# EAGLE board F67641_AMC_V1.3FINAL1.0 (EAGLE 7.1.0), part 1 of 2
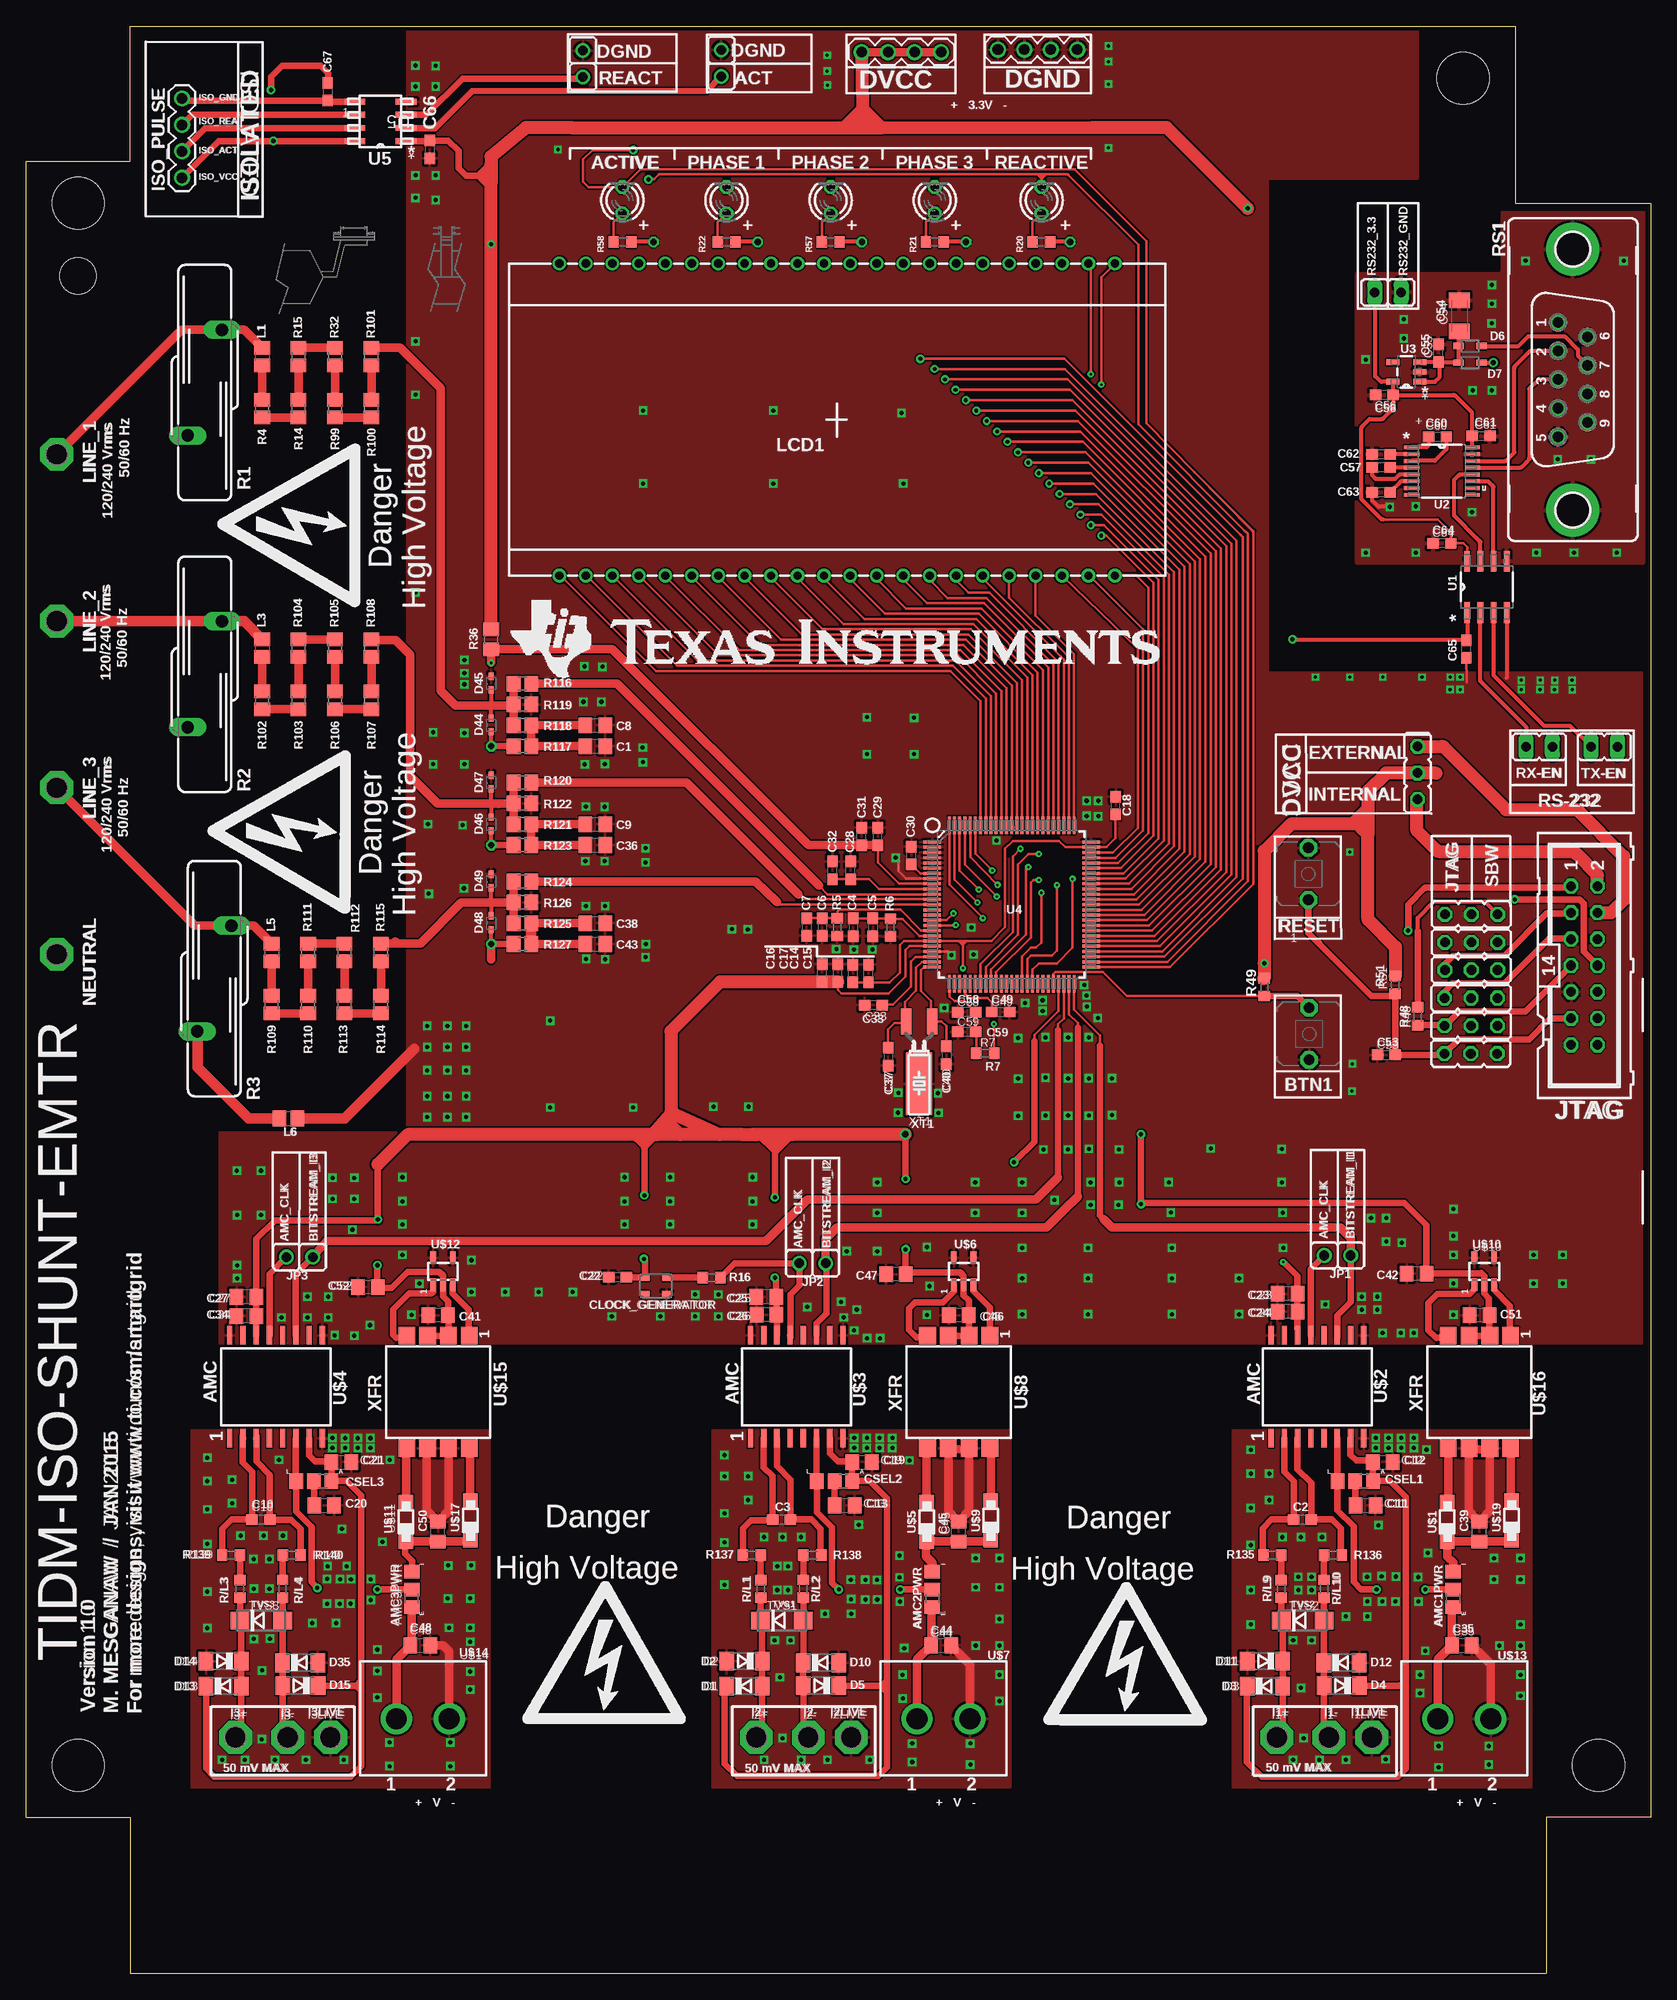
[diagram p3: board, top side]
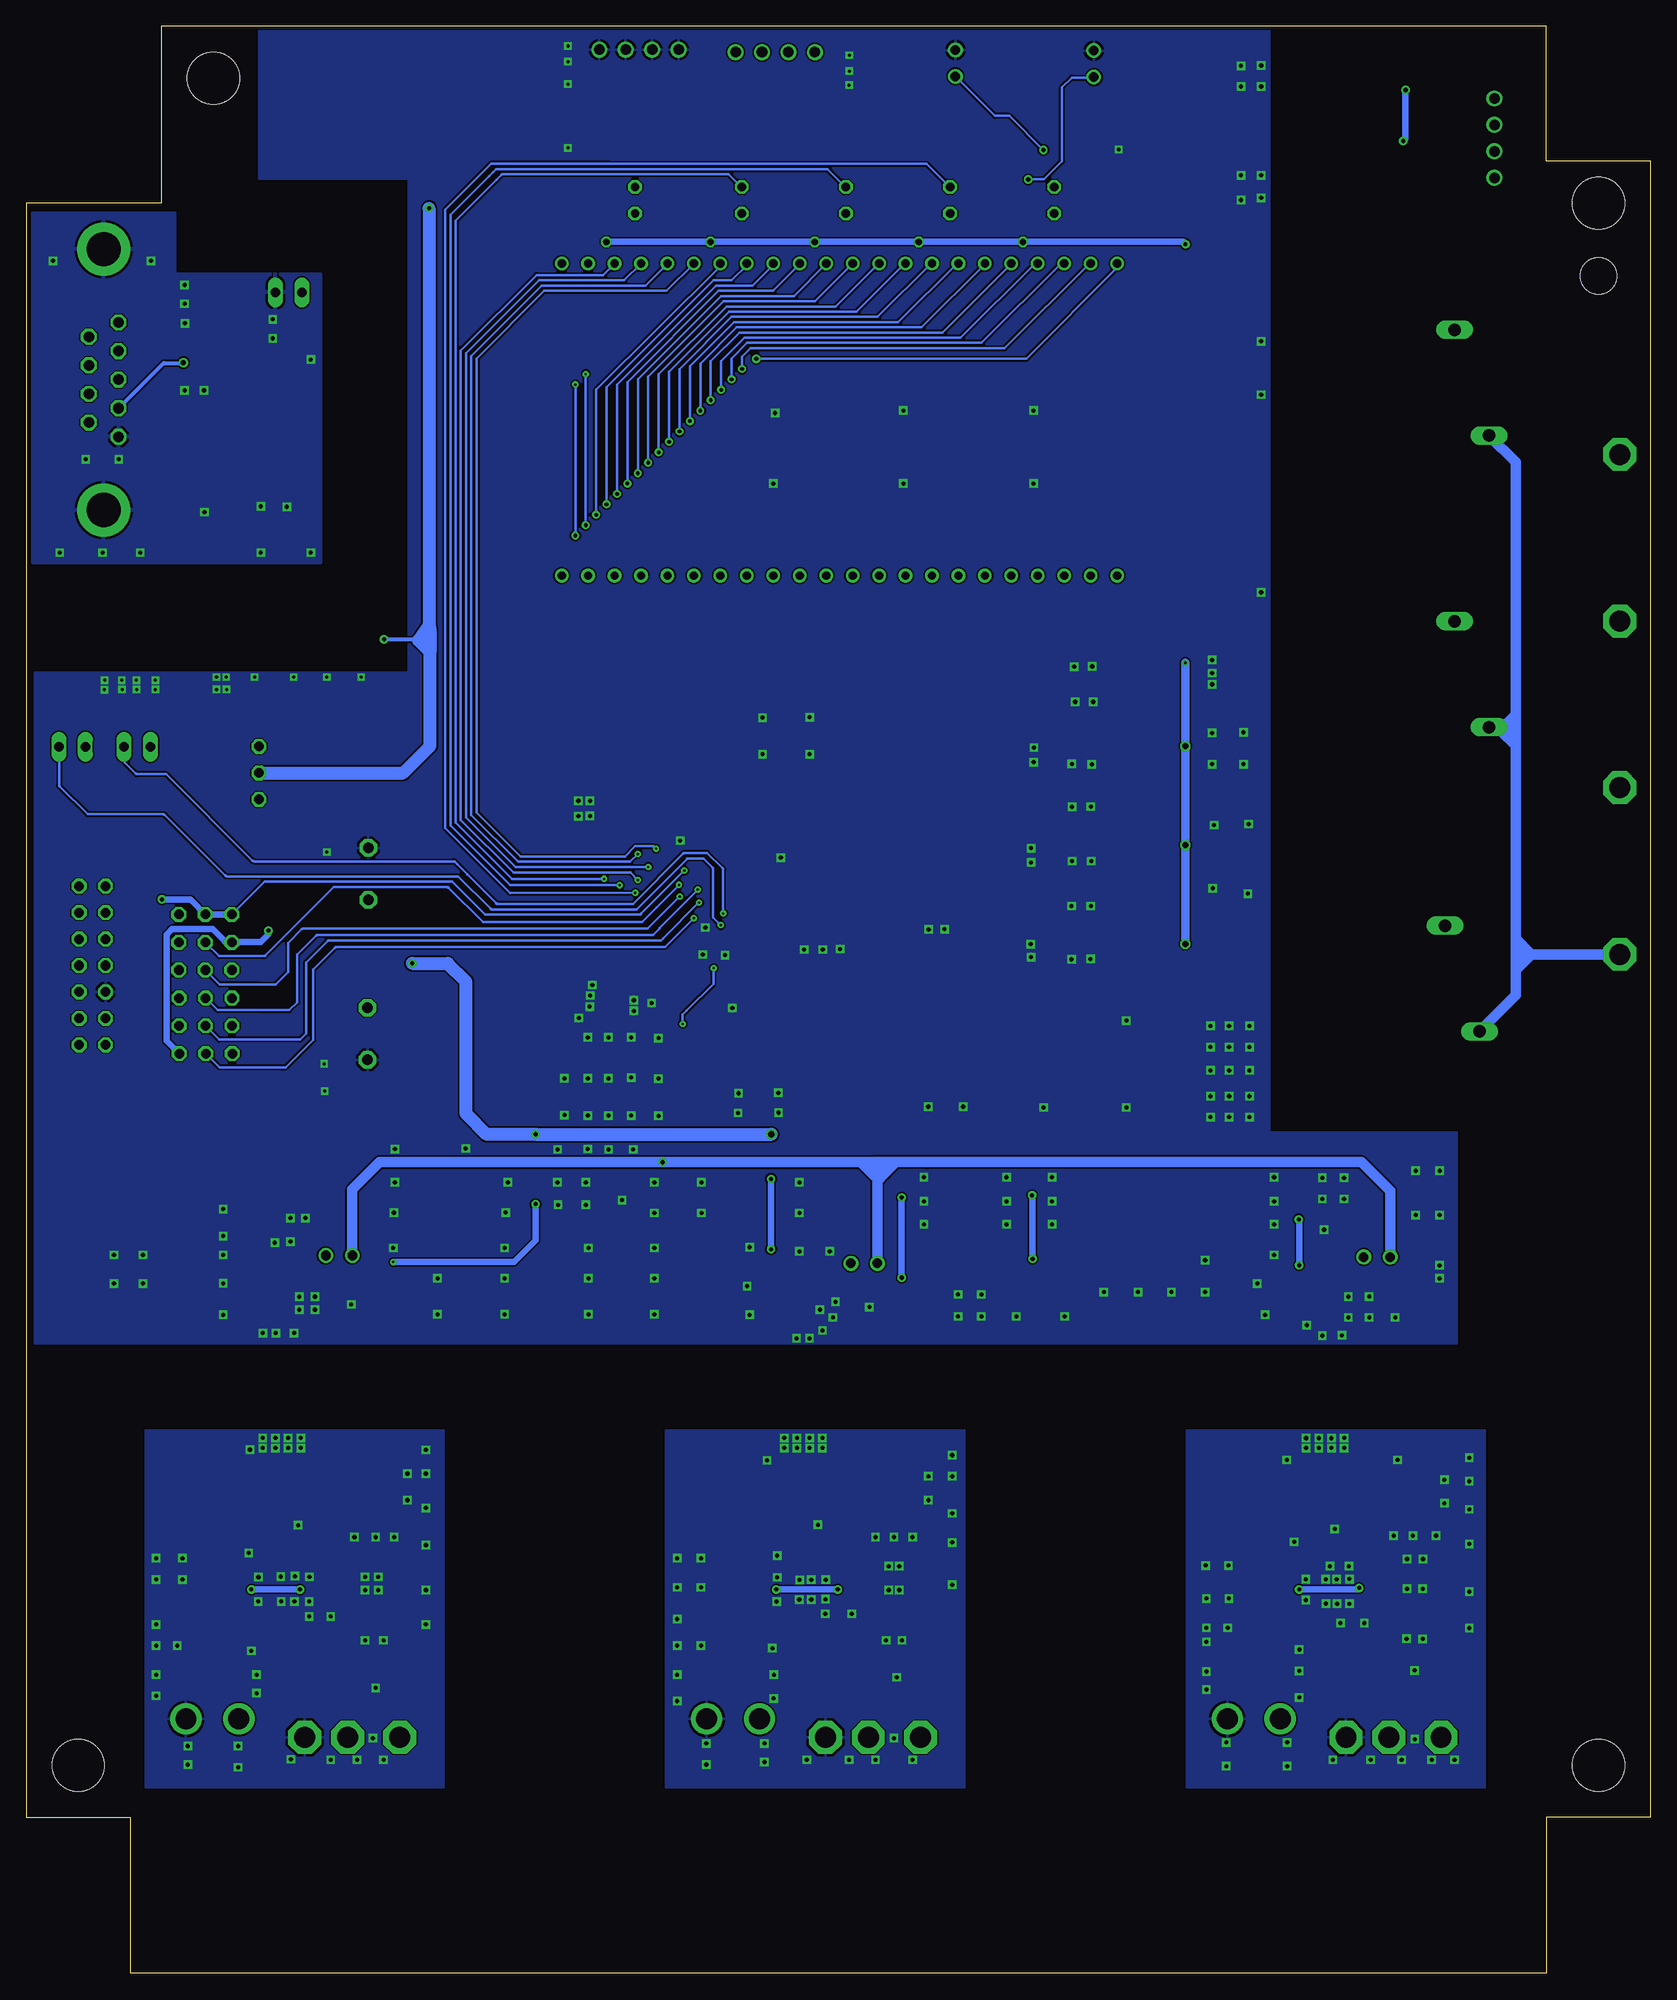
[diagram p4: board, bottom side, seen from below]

Size 156 x 187 mm. Coordinates in mm from the lower left corner, seen from the top.
Copper layers (1*16): Top 0.0356mm / dielectric 1.5011mm / Bottom 0.0356mm
Design rules "typical_4pcb *": minimum track width 10mil, minimum drill 0.2mm, track to track 6mil, track to pad 6mil, pad to pad 6mil, via to via 6mil, smd to smd 6mil, copper to edge 15mil, drill to drill 8mil, minimum pad ring 10mil, minimum via ring 8mil, stop-mask expansion 4mil, vias tented up to drill 25mil, thermal gap 10mil

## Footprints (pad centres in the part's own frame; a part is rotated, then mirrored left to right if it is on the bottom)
JP1 = drill 0.914: 1 0,-1.27; 2 0,1.27
A0R-JMP = smd 1.5 x 1.3: 1 0,1.7; 2 0,0; 3 0,-1.7
PBTH = drill 1.016 pad 1.676 octagon: 1 -0.001,0.001; 2 5.001,0.001
C0805 = smd 1.3 x 1.5: 1 -0.95,0; 2 0.95,0
C0603 = smd 1.1 x 1: 1 -0.85,0; 2 0.85,0
C1206K = smd 1.5 x 2: 1 -1.5,0; 2 1.5,0
3_PHASE_CASE = hole 5: 0,0; 146,0; 0,150; 133,162 | hole 3.5: 0,143
ASE = smd 0.9 x 0.65: 1 -1.05,-0.825; 2 1.05,-0.825; 3 1.05,0.825; 4 -1.05,0.825
SOD80C = smd 1.4 x 1.8: A 1.7,0; C -1.7,0
SOD323 = smd 1 x 0.6: 1 -1.1,0; 2 1.1,0
SOD523 = smd 0.7 x 0.5: A 0.7,0; C -0.6,0
MA04-1 = drill 1.016: 1 -3.81,0; 2 -1.27,0; 3 1.27,0; 4 3.81,0
P1-20 = drill 2.007 pad 3.15 octagon: TP 0,0
JP2 = drill 0.914 octagon: 1 -2.54,0; 2 0,0; 3 2.54,0
JP1' = drill 0.914 long: 1 0,-1.27; 2 0,1.27
ML14 = drill 0.914 octagon: 1 -7.62,-1.27; 2 -7.62,1.27; 3 -5.08,-1.27; 4 -5.08,1.27; 5 -2.54,-1.27; 6 -2.54,1.27; 7 0,-1.27; 8 0,1.27; 9 2.54,-1.27; 10 2.54,1.27; 11 5.08,-1.27; 12 5.08,1.27; 13 7.62,-1.27; 14 7.62,1.27
R0805 = smd 1.3 x 1.5: 1 -0.85,0; 2 0.85,0
TI_160SEG_LCD = drill 0.8: 1 4.826,0; 2 7.366,0; 3 9.906,0; 4 12.446,0; 5 14.986,0; 6 17.526,0; 7 20.066,0; 8 22.606,0; 9 25.146,0; 10 27.686,0; 11 30.226,0; 12 32.766,0; 13 35.306,0; 14 37.846,0; 15 40.386,0; 16 42.926,0; 17 45.466,0; 18 48.006,0; 19 50.546,0; 20 53.086,0; 21 55.626,0; 22 58.166,0; 23 58.166,29.972; 24 55.626,29.972; 29 42.926,29.972; 30 40.386,29.972; 31 37.846,29.972; 32 35.306,29.972; 33 32.766,29.972; 34 30.226,29.972; 35 27.686,29.972; 36 25.146,29.972; 37 22.606,29.972; 38 20.066,29.972; 39 17.526,29.972; 40 14.986,29.972; 41 12.446,29.972; 42 9.906,29.972; 43 7.366,29.972; 44 4.826,29.972; COM0 45.466,29.972; COM1 48.006,29.972; COM2 50.546,29.972; COM3 53.086,29.972
LED3MM = drill 0.813 octagon: A -1.27,0; K 1.27,0
S20K275 = drill 1.194 long: 1 -1.651,-5.08; 2 1.651,5.08
R0603 = smd 1 x 1.1: 1 -0.85,0; 2 0.85,0
R0805' = smd 1.3 x 1.5: 1 -0.95,0; 2 0.95,0
F09VP = drill 1.016 octagon: 1 5.486,1.422; 2 2.743,1.422; 3 0,1.422; 4 -2.743,1.422; 5 -5.486,1.422; 6 4.115,-1.422; 7 1.372,-1.422; 8 -1.372,-1.422; 9 -4.115,-1.422 | drill 3.302 pad 5.08: G1 -12.522,0; G2 12.522,0
DO214AC = smd 1.8 x 1.7: A 2.05,0; C -2.05,0
SOIC127P600X175-8N = smd 1.981 x 0.559: 1 -2.464,1.905; 2 -2.464,0.635; 3 -2.464,-0.635; 4 -2.464,-1.905; 5 2.464,-1.905; 6 2.464,-0.635; 7 2.464,0.635; 8 2.464,1.905
SOP65P640X120-16N = smd 1.473 x 0.356: 1 -2.921,2.286; 2 -2.921,1.626; 3 -2.921,0.965; 4 -2.921,0.33; 5 -2.921,-0.33; 6 -2.921,-0.965; 7 -2.921,-1.626; 8 -2.921,-2.286; 9 2.921,-2.286; 10 2.921,-1.626; 11 2.921,-0.965; 12 2.921,-0.33; 13 2.921,0.33; 14 2.921,0.965; 15 2.921,1.626; 16 2.921,2.286
SOT95P280X145-5N = smd 1.27 x 0.559: 1 -1.295,0.94; 2 -1.295,0; 3 -1.295,-0.94; 4 1.295,-0.94; 5 1.295,0.94
PZ100 = smd 1.676 x 0.279: 1 -7.62,5.994; 2 -7.62,5.512; 3 -7.62,5.004; 4 -7.62,4.496; 5 -7.62,3.988; 6 -7.62,3.505; 7 -7.62,2.997; 8 -7.62,2.489; 9 -7.62,2.007; 10 -7.62,1.499; 11 -7.62,0.991; 12 -7.62,0.508; 13 -7.62,0; 14 -7.62,-0.508; 15 -7.62,-0.991; 16 -7.62,-1.499; 17 -7.62,-2.007; 18 -7.62,-2.489; 19 -7.62,-2.997; 20 -7.62,-3.505; 21 -7.62,-3.988; 22 -7.62,-4.496; 23 -7.62,-5.004; 24 -7.62,-5.512; 25 -7.62,-5.994; 51 7.62,-5.994; 52 7.62,-5.512; 53 7.62,-5.004; 54 7.62,-4.496; 55 7.62,-3.988; 56 7.62,-3.505; 57 7.62,-2.997; 58 7.62,-2.489; 59 7.62,-2.007; 60 7.62,-1.499; 61 7.62,-0.991; 62 7.62,-0.508; 63 7.62,0; 64 7.62,0.508; 65 7.62,0.991; 66 7.62,1.499; 67 7.62,2.007; 68 7.62,2.489; 69 7.62,2.997; 70 7.62,3.505; 71 7.62,3.988; 72 7.62,4.496; 73 7.62,5.004; 74 7.62,5.512; 75 7.62,5.994 | smd 0.279 x 1.676: 26 -5.994,-7.62; 27 -5.512,-7.62; 28 -5.004,-7.62; 29 -4.496,-7.62; 30 -3.988,-7.62; 31 -3.505,-7.62; 32 -2.997,-7.62; 33 -2.489,-7.62; 34 -2.007,-7.62; 35 -1.499,-7.62; 36 -0.991,-7.62; 37 -0.508,-7.62; 38 0,-7.62; 39 0.508,-7.62; 40 0.991,-7.62; 41 1.499,-7.62; 42 2.007,-7.62; 43 2.489,-7.62; 44 2.997,-7.62; 45 3.505,-7.62; 46 3.988,-7.62; 47 4.496,-7.62; 48 5.004,-7.62; 49 5.512,-7.62; 50 5.994,-7.62; 76 5.994,7.62; 77 5.512,7.62; 78 5.004,7.62; 79 4.496,7.62; 80 3.988,7.62; 81 3.505,7.62; 82 2.997,7.62; 83 2.489,7.62; 84 2.007,7.62; 85 1.499,7.62; 86 0.991,7.62; 87 0.508,7.62; 88 0,7.62; 89 -0.508,7.62; 90 -0.991,7.62; 91 -1.499,7.62; 92 -2.007,7.62; 93 -2.489,7.62; 94 -2.997,7.62; 95 -3.505,7.62; 96 -3.988,7.62; 97 -4.496,7.62; 98 -5.004,7.62; 99 -5.512,7.62; 100 -5.994,7.62
D8 = smd 1.981 x 0.559: 1 -2.464,1.905; 2 -2.464,0.635; 3 -2.464,-0.635; 4 -2.464,-1.905; 5 2.464,-1.905; 6 2.464,-0.635; 7 2.464,0.635; 8 2.464,1.905
SOD123 = smd 1.4 x 1.4: A 1.9,0; C -1.9,0
SOIC-16DW = smd 1.778 x 0.508: AGND -5.029,-3.988; AINN -5.029,2.362; AINP -5.029,3.632; AVDD -5.029,-2.718; CLKIN 4.851,1.092; DGND1 4.851,-3.988; DGND2 4.851,4.902; DOUT 4.851,-1.448; DVDD 4.851,2.362; LDO_IN -5.029,-1.448; NC1 -5.029,4.902; NC2 -5.029,1.092; NC3 -5.029,-0.178; NC5 4.851,-2.718; NC6 4.851,-0.178; NC7 4.851,3.632
SOT23-DBV = smd 0.55 x 1.2: 1 -0.95,-1.3; 2 0,-1.3; 3 0.95,-1.3; 4 0.95,1.3; 5 -0.95,1.3
TERMINALBLOCK5.08 = drill 2: 1 -2.54,0; 2 2.54,0
DA2303-AL = smd 1.7 x 1.6: 1 -5.01,3.37; 2 -5.01,1.37; 3 -5.01,-0.63; 4 -5.01,-2.63; 5 5.79,-2.63; 6 5.79,-0.63; 7 5.79,1.37; 8 5.79,3.37
CM200T = smd 1 x 2.5: P1 -1.25,-5; P2 1.25,-5 | smd 2.5 x 6: P3 0,1

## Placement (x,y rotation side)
ACT  [JP1]  66.76,183.43 180 top
AMC1PWR  0R-JUMPA  [A0R-JMP]  137.04,36.87 180 top
AMC2PWR  0R-JUMPA  [A0R-JMP]  87.04,36.87 180 top
AMC3PWR  0R-JUMPA  [A0R-JMP]  37.04,36.87 180 top
BTN1  [PBTH]  123.22,87.73 90 top
C1  100nF  [C0805]  54.67,117.85 0 top
C2  5600pF  [C0603]  122.56,43.6 0 top
C3  5600pF  [C0603]  72.56,43.6 0 top
C4  4.7uF  [C0603]  79.43,100.45 270 top
C5  100nF  [C0603]  81.31,100.46 270 top
C6  4.7uF  [C0603]  76.46,100.5 270 top
C7  100nF  [C0603]  74.96,100.5 270 top
C8  10uF  [C0805]  54.67,119.85 0 top
C9  100nF  [C0805]  54.67,110.35 0 top
C10  5600pF  [C0603]  22.56,43.6 0 top
C11  0.1u  [C0805]  128.63,44.95 0 top
C12  4.7uF  [C0805]  130.28,49.11 0 top
C13  0.1u  [C0805]  78.63,44.95 0 top
C14  4.7uF  [C0603]  79.4,96.02 90 top
C15  100nF  [C0603]  80.9,96.02 90 top
C16  4.7uF  [C0603]  76.46,96.06 90 top
C17  100nF  [C0603]  77.96,96.06 90 top
C18  0.1uF  [C0603]  104.65,112.14 90 top
C19  4.7uF  [C0805]  80.28,49.11 0 top
C20  0.1u  [C0805]  28.63,44.95 0 top
C21  4.7uF  [C0805]  30.28,49.11 0 top
C22  0.01uF  [C0603]  56.81,66.86 180 top
C23  0.1u  [C0805]  121.14,65.27 180 top
C24  2.2uF  [C0805]  121.14,63.56 180 top
C25  0.1u  [C0805]  71.09,64.96 180 top
C26  2.2uF  [C0805]  71.11,63.26 180 top
C27  0.1u  [C0805]  21.16,64.96 180 top
C28  100nF  [C0603]  79.19,105.93 90 top
C29  4.7uF  [C0603]  81.79,109.18 90 top
C30  100nF  [C0603]  85.02,107.35 90 top
C31  100nF  [C0603]  80.24,109.18 90 top
C32  4.7uF  [C0603]  77.44,105.93 90 top
C33  470nF  [C0603]  81.38,92.98 180 top
C34  2.2uF  [C0805]  21.16,63.13 180 top
C35  10u  [C0805]  137.88,31.51 0 top
C36  10uF  [C0805]  54.67,108.35 0 top
C37  12pF  [C0603]  82.79,88.03 270 top
C38  100nF  [C0805]  54.67,100.85 0 top
C39  10u  [C0805]  139.55,42.43 90 top
C40  12pF  [C0603]  88.38,88.17 270 top
C41  10u  [C0805]  39.58,63.21 180 top
C42  0.1u  [C0805]  133.53,67.2 180 top
C43  10uF  [C0805]  54.67,98.85 0 top
C44  10u  [C0805]  87.88,31.51 0 top
C45  10u  [C0805]  89.55,42.43 90 top
C46  10u  [C0805]  89.58,63.21 180 top
C47  0.1u  [C0805]  83.53,67.15 180 top
C48  10u  [C0805]  37.88,31.51 0 top
C49  4.7uF  [C0603]  93.59,92.32 0 top
C50  10u  [C0805]  39.55,42.43 90 top
C51  10u  [C0805]  139.58,63.21 180 top
C52  0.1u  [C0805]  32.82,65.9 180 top
C53  0.1uF  [C0603]  130.64,88.2 0 top
C54  47u  [C1206K]  137.65,159.17 90 top
C55  1u  [C0603]  135.64,155.59 90 top
C56  0.1u  [C0603]  130.43,151.58 180 top
C57  0.1u  [C0603]  130.13,144.62 180 top
C58  0.47uF  [C0603]  90.33,92.32 180 top
C59  100nF  [C0603]  90.33,90.41 180 top
C60  0.1u  [C0603]  135.54,147.56 0 top
C61  0.1u  [C0603]  139.73,147.64 0 top
C62  0.1u  [C0603]  130.13,145.89 0 top
C63  0.1u  [C0603]  130.13,142.23 0 top
C64  0.1u  [C0603]  135.97,137.33 180 top
C65  0.1u  [C0603]  138.31,127.17 90 top
C66  0.1u  [C0603]  38.76,175.15 270 top
C67  0.1u  [C0603]  28.96,180.68 270 top
CASE1  3_PHASE_CASE  [3_PHASE_CASE]  5,20 0 top
CLOCK_GENERATOR  ASE  [ASE]  60.48,66.02 0 top
CSEL1  0R-JUMPA  [A0R-JMP]  127.64,47.28 270 top
CSEL2  0R-JUMPA  [A0R-JMP]  77.64,47.28 270 top
CSEL3  0R-JUMPA  [A0R-JMP]  27.64,47.28 270 top
D1  PMLL4148  [SOD80C]  68.98,27.59 0 top
D2  PMLL4148  [SOD80C]  68.98,29.99 180 top
D3  PMLL4148  [SOD80C]  118.98,27.59 0 top
D4  PMLL4148  [SOD80C]  126.35,27.64 180 top
D5  PMLL4148  [SOD80C]  76.35,27.64 180 top
D6  1N4148  [SOD323]  138.66,156.27 0 top
D7  1N4148  [SOD323]  138.66,154.67 0 top
D10  PMLL4148  [SOD80C]  76.32,29.84 0 top
D11  PMLL4148  [SOD80C]  118.98,29.99 180 top
D12  PMLL4148  [SOD80C]  126.32,29.84 0 top
D13  PMLL4148  [SOD80C]  18.98,27.59 0 top
D14  PMLL4148  [SOD80C]  18.98,29.99 180 top
D15  PMLL4148  [SOD80C]  26.35,27.64 180 top
D35  PMLL4148  [SOD80C]  26.32,29.84 0 top
D44  1N4148DO35-7  [SOD523]  44.67,119.85 90 top
D45  1N4148DO35-7  [SOD523]  44.67,123.85 90 top
D46  1N4148DO35-7  [SOD523]  44.67,110.35 90 top
D47  1N4148DO35-7  [SOD523]  44.67,114.35 90 top
D48  1N4148DO35-7  [SOD523]  44.67,100.85 90 top
D49  1N4148DO35-7  [SOD523]  44.67,104.85 90 top
DGND  [MA04-1]  97.14,184.73 0 top
DVCC  [MA04-1]  84.05,184.5 0 top
I1+  TPPAD1-20  [P1-20]  120.12,22.67 0 top
I1-  TPPAD1-20  [P1-20]  125.12,22.67 0 top
I1LIVE  TPPAD1-20  [P1-20]  129.24,22.67 0 top
I2+  TPPAD1-20  [P1-20]  70.12,22.67 0 top
I2-  TPPAD1-20  [P1-20]  75.12,22.67 0 top
I2LIVE  TPPAD1-20  [P1-20]  79.24,22.67 0 top
I3+  TPPAD1-20  [P1-20]  20.12,22.67 0 top
I3-  TPPAD1-20  [P1-20]  25.12,22.67 0 top
I3LIVE  TPPAD1-20  [P1-20]  29.24,22.67 0 top
ISO_PULSE  [MA04-1]  14.99,176.24 90 top
JP1  [JP1]  125.94,68.95 90 top
JP2  [JP1]  75.52,68.19 90 top
JP3  [JP1]  26.27,68.8 90 top
JP4  [JP2]  138.79,101.69 180 top
JP5  [JP2]  138.74,88.33 180 top
JP6  [JP2]  138.76,91 180 top
JP7  [JP2]  138.76,93.66 180 top
JP8  [JP2]  138.79,96.36 180 top
JP9  [JP2]  138.79,99 180 top
JP10  [JP2]  133.63,115.28 90 top
JP14  [JP1']  130.79,161.43 270 top
JP15  [JP1']  145.32,117.79 90 top
JP16  [JP1']  151.57,117.79 90 top
JTAG  [ML14]  149.64,96.79 270 top
L1  EXCML20A  [R0805]  22.67,155.26 270 top
L3  EXCML20A  [R0805]  22.67,127.26 270 top
L5  EXCML20A  [R0805]  23.59,98.04 270 top
L6  EXCML20A  [R0805]  25.2,82.1 0 top
LCD1  TI_160SEG_LCD  [TI_160SEG_LCD]  46.4,134.23 0 top
LED_ACT  [LED3MM]  57.27,170.27 90 top
LED_PHASE_1  [LED3MM]  67.27,170.27 90 top
LED_PHASE_2  [LED3MM]  77.27,170.27 90 top
LED_PHASE_3  [LED3MM]  87.27,170.27 90 top
LED_REACT  [LED3MM]  97.52,170.27 90 top
LINE_1  TPPAD1-20  [P1-20]  2.96,145.86 0 top
LINE_2  TPPAD1-20  [P1-20]  2.96,129.86 0 top
LINE_3  TPPAD1-20  [P1-20]  2.96,113.86 0 top
NEUTRAL  TPPAD1-20  [P1-20]  2.96,97.86 0 top
R1  S20K275  [S20K275]  17.17,152.76 0 top
R2  S20K275  [S20K275]  17.17,124.76 0 top
R3  S20K275  [S20K275]  18.09,95.54 0 top
R4  1M  [R0805]  22.67,150.26 90 top
R5  0  [R0603]  77.88,100.47 90 top
R6  0  [R0603]  83.01,100.44 90 top
R7  0  [R0603]  92.1,88.38 180 top
R14  1M  [R0805]  26.17,150.26 270 top
R15  1M  [R0805]  26.17,155.26 270 top
R16  0  [R0603]  65.83,66.81 0 top
R20  100  [R0603]  97.52,166.27 180 top
R21  100  [R0603]  87.27,166.27 180 top
R22  100  [R0603]  67.27,166.27 180 top
R32  1M  [R0805]  29.67,155.26 90 top
R36  10R  [R0805']  44.66,128.11 270 top
R48  330  [R0603]  133.63,91.91 90 top
R49  100K  [R0603]  118.91,94.71 270 top
R51  47K  [R0603]  131.47,94.93 270 top
R57  100  [R0603]  77.27,166.27 180 top
R58  100  [R0603]  57.27,166.27 180 top
R99  1M  [R0805]  29.67,150.26 90 top
R100  1M  [R0805]  33.17,150.26 270 top
R101  1M  [R0805]  33.17,155.26 270 top
R102  1M  [R0805]  22.67,122.26 90 top
R103  1M  [R0805]  26.17,122.26 270 top
R104  1M  [R0805]  26.17,127.26 270 top
R105  1M  [R0805]  29.67,127.26 90 top
R106  1M  [R0805]  29.67,122.26 90 top
R107  1M  [R0805]  33.17,122.26 270 top
R108  1M  [R0805]  33.17,127.26 270 top
R109  1M  [R0805]  23.59,93.04 90 top
R110  1M  [R0805]  27.09,93.04 270 top
R111  1M  [R0805]  27.09,98.04 270 top
R112  1M  [R0805]  30.59,98.04 90 top
R113  1M  [R0805]  30.59,93.04 90 top
R114  1M  [R0805]  34.09,93.04 270 top
R115  1M  [R0805]  34.09,98.04 270 top
R116  1K  [R0805]  47.67,123.85 0 top
R117  10  [R0805]  47.67,117.85 0 top
R118  20K  [R0805]  47.67,119.85 180 top
R119  10K  [R0805]  47.67,121.85 180 top
R120  1K  [R0805]  47.67,114.35 0 top
R121  20K  [R0805]  47.67,110.35 180 top
R122  10K  [R0805]  47.67,112.35 180 top
R123  10  [R0805]  47.67,108.35 0 top
R124  1K  [R0805]  47.67,104.85 0 top
R125  20K  [R0805]  47.67,100.85 180 top
R126  10K  [R0805]  47.67,102.85 180 top
R127  10  [R0805]  47.67,98.85 0 top
R135  20.0  [R0603]  119.69,40.17 0 top
R136  20.0  [R0603]  125.51,40.17 180 top
R137  20.0  [R0603]  69.69,40.17 0 top
R138  20.0  [R0603]  75.51,40.17 180 top
R139  20.0  [R0603]  19.69,40.17 0 top
R140  20.0  [R0603]  25.51,40.17 180 top
R/L1  0  [R0603]  70.54,36.92 270 top
R/L2  0  [R0603]  74.64,36.95 270 top
R/L3  0  [R0603]  20.54,36.92 270 top
R/L4  0  [R0603]  24.64,36.95 270 top
R/L9  0  [R0603]  120.54,36.92 270 top
R/L10  0  [R0603]  124.64,36.95 270 top
REACT  [JP1]  53.47,183.38 180 top
RESET  [PBTH]  123.14,103.09 90 top
RS1  [F09VP]  148.54,153.05 90 top
TVS1  SMAJ5.0CA  [DO214AC]  72.59,33.89 0 top
TVS2  SMAJ5.0CA  [DO214AC]  122.59,33.89 0 top
TVS3  SMAJ5.0CA  [DO214AC]  22.59,33.89 0 top
U1  ISO7421D  [SOIC127P600X175-8N]  140.29,133.13 90 top
U2  TRS3232EQPWRQ1  [SOP65P640X120-16N]  135.97,144.26 0 top
U3  TPS76333DBVT  [SOT95P280X145-5N]  132.54,153.78 180 top
U4  MSP430F67641_PZ_100  [PZ100]  94.66,102.64 0 top
U5  ISO7420_D_8  [D8]  34.04,177.84 180 top
U$1  DIODE-SCHOTTKY-CUSTOM  [SOD123]  136.48,43.37 90 top
U$2  AMC  [SOIC-16DW]  124.46,56.43 90 top
U$3  AMC  [SOIC-16DW]  74.46,56.43 90 top
U$4  AMC  [SOIC-16DW]  24.46,56.43 90 top
U$5  DIODE-SCHOTTKY-CUSTOM  [SOD123]  86.48,43.37 90 top
U$6  SN6501  [SOT23-DBV]  90.03,67.42 0 top
U$7  CUSTOM_TERMINAL_BLOCK  [TERMINALBLOCK5.08]  88.1,24.45 0 top
U$8  CUSTOM_TRANSFORMER_AMC  [DA2303-AL]  89.2,56.22 270 top
U$9  DIODE-SCHOTTKY-CUSTOM  [SOD123]  92.65,43.5 90 top
U$10  SN6501  [SOT23-DBV]  140.03,67.42 0 top
U$11  DIODE-SCHOTTKY-CUSTOM  [SOD123]  36.48,43.37 90 top
U$12  SN6501  [SOT23-DBV]  40.03,67.42 0 top
U$13  CUSTOM_TERMINAL_BLOCK  [TERMINALBLOCK5.08]  138.1,24.45 0 top
U$14  CUSTOM_TERMINAL_BLOCK  [TERMINALBLOCK5.08]  38.1,24.45 0 top
U$15  CUSTOM_TRANSFORMER_AMC  [DA2303-AL]  39.2,56.22 270 top
U$16  CUSTOM_TRANSFORMER_AMC  [DA2303-AL]  139.2,56.22 270 top
U$17  DIODE-SCHOTTKY-CUSTOM  [SOD123]  42.65,43.5 90 top
U$19  DIODE-SCHOTTKY-CUSTOM  [SOD123]  142.65,43.5 90 top
XT1  [CM200T]  85.75,86.41 180 top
